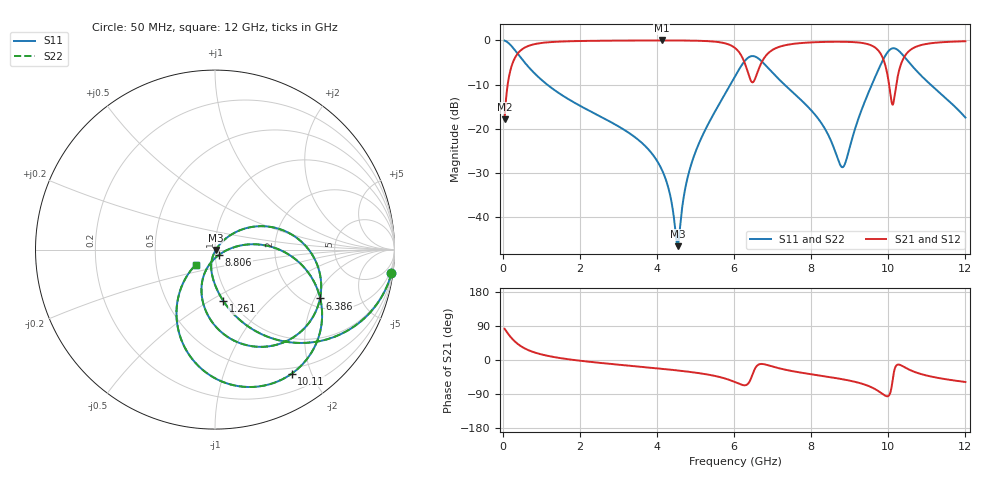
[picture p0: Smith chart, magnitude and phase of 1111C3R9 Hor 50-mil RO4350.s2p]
# GHz S MA R 50
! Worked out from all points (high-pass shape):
!   11951 points, 50 MHz to 12 GHz, reference 50 ohm
!   highest |S21| = -0.04 dB at 4.123 GHz (marker M1); lowest = -17.9 dB at 50 MHz (marker M2)
!   |S21| within 3 dB of the highest: 386.2 MHz to 6.159 GHz (5.773 GHz wide, 176 % of centre); 6.872 GHz to 9.803 GHz (2.931 GHz wide, 35.2 % of centre)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
!   lowest |S11| = -46.5 dB at 4.535 GHz (marker M3), VSWR 1.01, Z = 50.4 - j0.242 ohm
!   |S11| at or under -10 dB: 1.154 GHz to 5.903 GHz (4.748 GHz wide, 135 % of centre); 7.307 GHz to 9.574 GHz (2.267 GHz wide, 26.9 % of centre); 11.1 GHz to end of sweep
!   |S22| runs from -46.5 to -0.1 dB; largest |S21 - S12| = 0
!   S11 on the Smith chart (normalised r, x): 50 MHz: 1, -15; 1.261 GHz: 0.92, -0.58; 6.386 GHz: 2.37, -2.21; 8.806 GHz: 1.04, -0.06; 10.11 GHz: 0.42, -1.72; 12 GHz: 0.80, -0.14
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0.05  0.9918 -7.6  0.1277 82.3  0.1277 82.3  0.9918 -7.6
0.185  0.9027 -26.6  0.4301 63.4  0.4301 63.4  0.9027 -26.6
0.365  0.7282 -45.5  0.6848 44.5  0.6848 44.5  0.7282 -45.5
0.714  0.4765 -65.9  0.8783 24.0  0.8783 24.0  0.4765 -65.9
1.261  0.2912 -80.7  0.9555 9.1  0.9555 9.1  0.2912 -80.7
2.042  0.1787 -91.9  0.9824 -2.3  0.9824 -2.3  0.1787 -91.9
4.034  0.04141 -108.1  0.9959 -22.3  0.9959 -22.3  0.04141 -108.1
4.123  0.03495 -107.9  0.9959 -23.2  0.9959 -23.2  0.03495 -107.9
4.535  0.004742 -30.4  0.995 -27.6  0.995 -27.6  0.004742 -30.4
4.959  0.04903 47.6  0.9904 -32.8  0.9904 -32.8  0.04903 47.6
6.025  0.3926 16.0  0.8192 -58.3  0.8192 -58.3  0.3926 16.0
6.386  0.6453 -24.9  0.3991 -59.6  0.3991 -59.6  0.6453 -24.9
6.636  0.6213 -59.8  0.4696 -12.1  0.4696 -12.1  0.6213 -59.8
7.005  0.4274 -89.6  0.7825 -17.4  0.7825 -17.4  0.4274 -89.6
8.017  0.1594 -113.4  0.9478 -37.9  0.9478 -37.9  0.1594 -113.4
8.806  0.03691 -55.1  0.9627 -50.6  0.9627 -50.6  0.03691 -55.1
9.635  0.3641 -0.4  0.8418 -75.5  0.8418 -75.5  0.3641 -0.4
10.009  0.7581 -40.7  0.3424 -94.4  0.3424 -94.4  0.7581 -40.7
10.114  0.8126 -58.3  0.1876 -52.5  0.1876 -52.5  0.8126 -58.3
10.337  0.7138 -90.4  0.5485 -14.4  0.5485 -14.4  0.7138 -90.4
10.591  0.5302 -111.1  0.7888 -27.6  0.7888 -27.6  0.5302 -111.1
12  0.1342 -141.8  0.9758 -58.1  0.9758 -58.1  0.1342 -141.8
